(* Logix 5000 AddOnInstructionDefinition export AMCI_NXFE2_Encoder_Follower_CCW; software revision 20.03 *)

ADD_ON_INSTRUCTION AMCI_NXFE2_Encoder_Follower_CCW   (* revision 1.0, vendor AMCI, ExecuteEnableInFalse *)
VAR_INPUT
   Axis_Status_Bits : INT; {required}
   _0_normal_1_S_curve_acceleration : BOOL;
   _0_Triangular_1_Trapezoidal_S_Curve : BOOL;
   Encoder_Count_Multiplier : INT; {required}
   Encoder_count_Divisor : INT; {required}
   Acceleration : INT; {required}
   Deceleration : INT; {required}
END_VAR
VAR_IN_OUT
   NXFE2_output_data : _000A:NXFE2_0986AEB4:O:0; {required}
END_VAR
VAR_OUTPUT
   EN : BOOL; {access Read Only, visible}
   Encoder_Follower_Occurring : BOOL; {access Read Only, visible}
   ER : BOOL; {access Read Only, visible}
END_VAR
VAR
   command_data_block : INT[10];
        [0]   // Command Bits MSW
        [1]   // Command Bits LSW
        [4]   // Upper Programmed Speed
        [5]   // Lower Programmed Speed
END_VAR

ROUTINE EnableInFalse   (* ladder *)
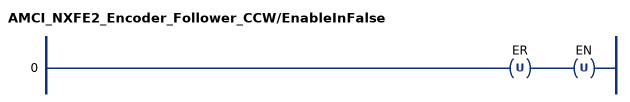
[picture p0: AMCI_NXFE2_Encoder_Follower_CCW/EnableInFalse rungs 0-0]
   0: OTU(ER)OTU(EN);
END_ROUTINE

ROUTINE Logic   (* ladder *)
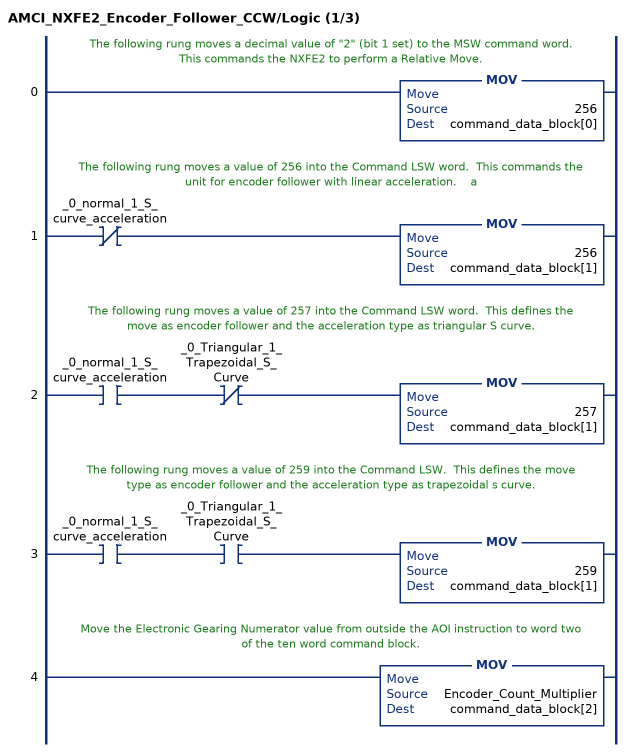
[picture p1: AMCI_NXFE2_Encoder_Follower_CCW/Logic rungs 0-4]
   // The following rung moves a decimal value of "2" (bit 1 set) to the MSW command word.  This commands the NXFE2 to perform a Relative Move.
   0: MOV(256,command_data_block[0]);
   // The following rung moves a value of 256 into the Command LSW word.  This commands the unit for encoder follower with linear acceleration.    a
   1: XIO(_0_normal_1_S_curve_acceleration)MOV(256,command_data_block[1]);
   // The following rung moves a value of 257 into the Command LSW word.  This defines the move as encoder follower and the acceleration type as triangular S curve.
   2: XIC(_0_normal_1_S_curve_acceleration)XIO(_0_Triangular_1_Trapezoidal_S_Curve)MOV(257,command_data_block[1]);
   // The following rung moves a value of 259 into the Command LSW.  This defines the move type as encoder follower and the acceleration type as trapezoidal s curve.
   3: XIC(_0_normal_1_S_curve_acceleration)XIC(_0_Triangular_1_Trapezoidal_S_Curve)MOV(259,command_data_block[1]);
   // Move the Electronic Gearing Numerator value from outside the AOI instruction to word two of the ten word command block.
   4: MOV(Encoder_Count_Multiplier,command_data_block[2]);
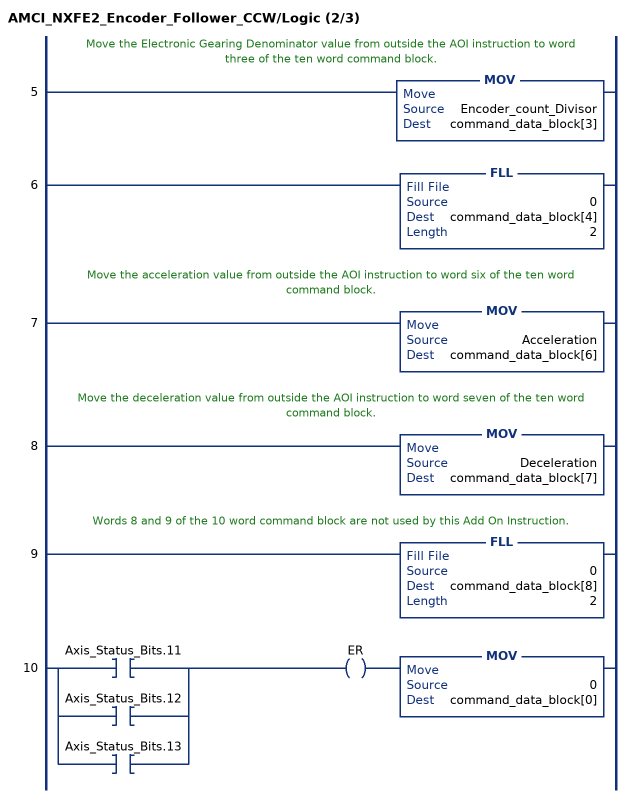
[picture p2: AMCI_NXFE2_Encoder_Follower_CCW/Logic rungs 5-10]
   // Move the Electronic Gearing Denominator value from outside the AOI instruction to word three of the ten word command block.
   5: MOV(Encoder_count_Divisor,command_data_block[3]);
   6: FLL(0,command_data_block[4],2);
   // Move the acceleration value from outside the AOI instruction to word six of the ten word command block.
   7: MOV(Acceleration,command_data_block[6]);
   // Move the deceleration value from outside the AOI instruction to word seven of the ten word command block.
   8: MOV(Deceleration,command_data_block[7]);
   // Words 8 and 9 of the 10 word command block are not used by this Add On Instruction.
   9: FLL(0,command_data_block[8],2);
   10: [XIC(Axis_Status_Bits.11) ,XIC(Axis_Status_Bits.12) ,XIC(Axis_Status_Bits.13) ]OTE(ER)MOV(0,command_data_block[0]);
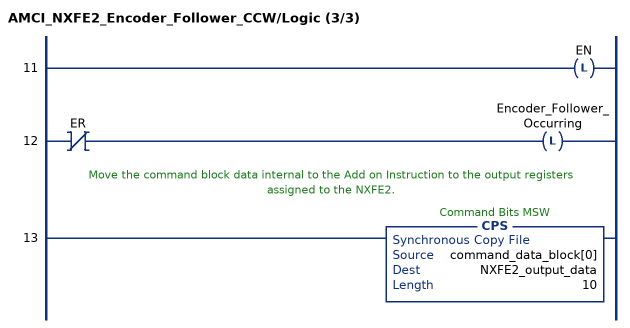
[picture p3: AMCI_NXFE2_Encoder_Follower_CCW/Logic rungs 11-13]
   11: OTL(EN);
   12: XIO(ER)OTL(Encoder_Follower_Occurring);
   // Move the command block data internal to the Add on Instruction to the output registers assigned to the NXFE2.
   13: CPS(command_data_block[0],NXFE2_output_data,10);
END_ROUTINE
END_ADD_ON_INSTRUCTION
